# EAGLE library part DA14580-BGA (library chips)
WLCSP package of low power BLE chip
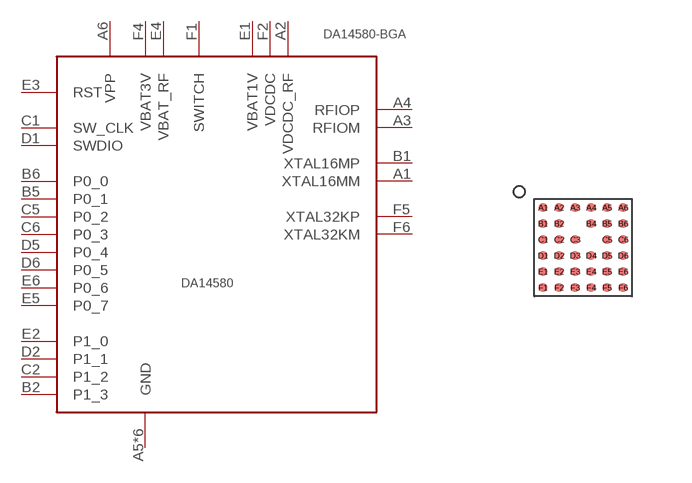
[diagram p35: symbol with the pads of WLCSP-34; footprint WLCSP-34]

Designator prefix -

## DA14580-BGA (DIGIKEY: 1564-1012-1-ND)  [WLCSP-34]
A1  XTAL16MM
A2  VDCDC_RF
A3  RFIOM
A4  RFIOP
A5  GND
A6  VPP
B1  XTAL16MP
B2  P1_3
B4  GND
B5  P0_1
B6  P0_0
C1  SW_CLK
C2  P1_2
C3  GND
C5  P0_2
C6  P0_3
D1  SWDIO
D2  P1_1
D3  GND
D4  GND
D5  P0_4
D6  P0_5
E1  VBAT1V
E2  P1_0
E3  RST
E4  VBAT_RF
E5  P0_7
E6  P0_6
F1  SWITCH
F2  VDCDC
F3  GND
F4  VBAT3V
F5  XTAL32KP
F6  XTAL32KM

## Footprint WLCSP-34 (pad centres in mm)
smd 0.22 x 0.22: A1 0,2; A2 0.4,2; A3 0.8,2; A4 1.2,2; A5 1.6,2; A6 2,2; B1 0,1.6; B2 0.4,1.6; B4 1.2,1.6; B5 1.6,1.6; B6 2,1.6; C1 0,1.2; C2 0.4,1.2; C3 0.8,1.2; C5 1.6,1.2; C6 2,1.2; D1 0,0.8; D2 0.4,0.8; D3 0.8,0.8; D4 1.2,0.8; D5 1.6,0.8; D6 2,0.8; E1 0,0.4; E2 0.4,0.4; E3 0.8,0.4; E4 1.2,0.4; E5 1.6,0.4; E6 2,0.4; F1 0,0; F2 0.4,0; F3 0.8,0; F4 1.2,0; F5 1.6,0; F6 2,0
